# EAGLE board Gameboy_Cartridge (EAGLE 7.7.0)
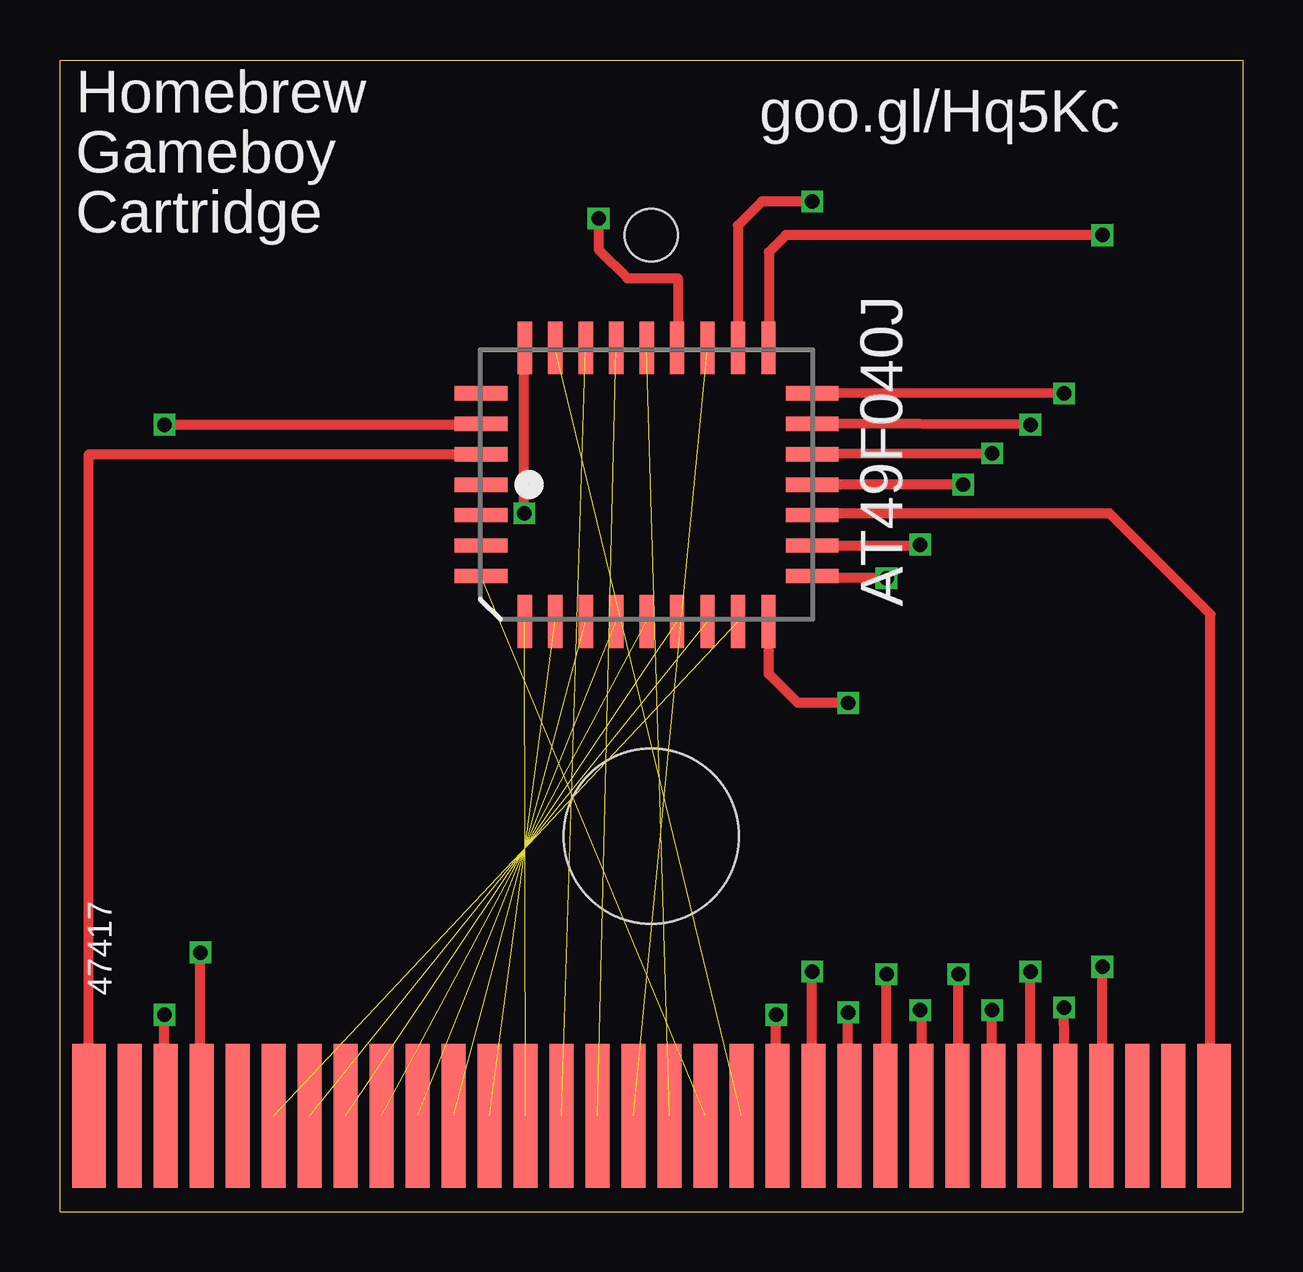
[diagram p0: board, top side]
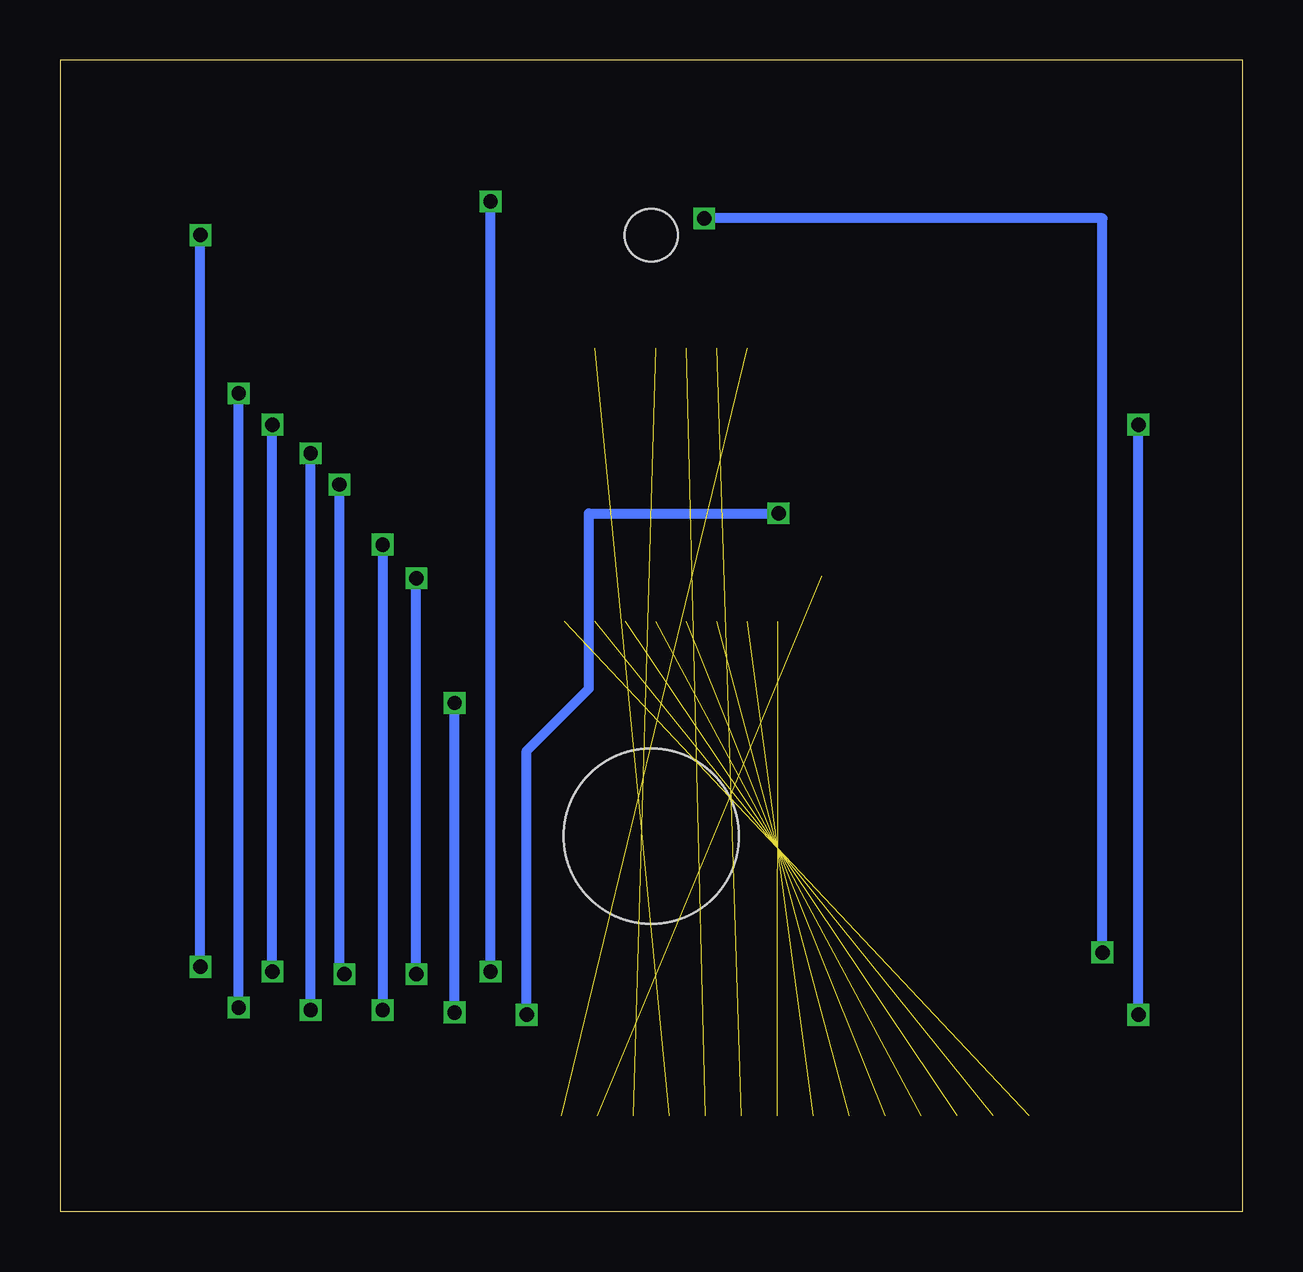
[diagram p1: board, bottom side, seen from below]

Size 49.3 x 48 mm. Coordinates in mm from the lower left corner, seen from the top.
Outline: 49.3,48 49.3,0 0,0 0,48 49.3,48
Copper layers (1*16): Top 0.035mm / dielectric 1.5mm / Bottom 0.035mm
Design rules "default": minimum track width 6mil, minimum drill 12mil, track to track 6mil, track to pad 6mil, pad to pad 6mil, via to via 6mil, smd to smd 0mil, copper to edge 10mil, drill to drill 10mil, minimum pad ring 10mil, minimum via ring 6mil, stop-mask expansion 2mil, vias tented up to drill 100mil, thermal gap 10mil
Holes 7.3 mm at 24.65,15.65
Holes 2.2 mm at 24.65,40.7

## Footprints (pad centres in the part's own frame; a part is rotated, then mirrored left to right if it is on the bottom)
PLCC32R = smd 0.6 x 2.2: 1 0,6.9; 2 -1.27,6.9; 3 -2.54,6.9; 4 -3.81,6.9; 14 -3.81,-6.9; 15 -2.54,-6.9; 16 -1.27,-6.9; 17 0,-6.9; 18 1.27,-6.9; 19 2.54,-6.9; 20 3.81,-6.9; 30 3.81,6.9; 31 2.54,6.9; 32 1.27,6.9 | smd 2.2 x 0.6: 5 -5.7,5.08; 6 -5.7,3.81; 7 -5.7,2.54; 8 -5.7,1.27; 9 -5.7,0; 10 -5.7,-1.27; 11 -5.7,-2.54; 12 -5.7,-3.81; 13 -5.7,-5.08; 21 5.7,-5.08; 22 5.7,-3.81; 23 5.7,-2.54; 24 5.7,-1.27; 25 5.7,0; 26 5.7,1.27; 27 5.7,2.54; 28 5.7,3.81; 29 5.7,5.08
CONNECTOR = smd 1.4 x 6: 1 0.7,-3; 32 47.6,-3 | smd 1 x 6: 2 2.4,-3; 3 3.9,-3; 4 5.4,-3; 5 6.9,-3; 6 8.4,-3; 7 9.9,-3; 8 11.4,-3; 9 12.9,-3; 10 14.4,-3; 11 15.9,-3; 12 17.4,-3; 13 18.9,-3; 14 20.4,-3; 15 21.9,-3; 16 23.4,-3; 17 24.9,-3; 18 26.4,-3; 19 27.9,-3; 20 29.4,-3; 21 30.9,-3; 22 32.4,-3; 23 33.9,-3; 24 35.4,-3; 25 36.9,-3; 26 38.4,-3; 27 39.9,-3; 28 41.4,-3; 29 42.9,-3; 30 44.4,-3; 31 45.9,-3

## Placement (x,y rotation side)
IC1  AT49F040J  [PLCC32R]  24.45,30.3 90 top
U$1  CONNECTOR  [CONNECTOR]  0.5,7 0 top

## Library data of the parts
IC1 U$1 = gameboy

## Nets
3: U$1.3
4: IC1.24 U$1.4
5: U$1.5
6: IC1.12 U$1.6
7: IC1.11 U$1.7
8: IC1.10 U$1.8
9: IC1.9 U$1.9
10: IC1.8 U$1.10
11: IC1.7 U$1.11
12: IC1.6 U$1.12
13: IC1.5 U$1.13
14: IC1.27 U$1.14
15: IC1.26 U$1.15
16: IC1.23 U$1.16
17: IC1.25 U$1.17
18: IC1.4 U$1.18
19: IC1.28 U$1.19
20: IC1.29 U$1.20
21: IC1.22 U$1.21
22: IC1.13 U$1.22
23: IC1.14 U$1.23
24: IC1.15 U$1.24
25: IC1.17 U$1.25
26: IC1.18 U$1.26
27: IC1.19 U$1.27
28: IC1.20 U$1.28
29: IC1.21 U$1.29
30: U$1.30
31: U$1.31
GND: IC1.16 U$1.32
S$1: IC1.31
VDD: IC1.32 U$1.1

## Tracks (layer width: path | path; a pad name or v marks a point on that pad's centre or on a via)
3  (via drill 0.6)
  Top 0.406: U$1.3 4.35,4 v4.35,8.2
  Bottom 0.406: v4.35,8.2 4.35,32.8
4  (via drill 0.6)
  Top 0.406: U$1.4 5.85,4 v5.85,10.8 | v22.45,41.4 22.45,40.1 23.65,38.9 25.75,38.9 25.75,36.03 IC1.24
  Bottom 0.406: v5.85,10.8 5.85,41.4 v22.45,41.4
6  (1 unrouted)
7  (1 unrouted)
8  (1 unrouted)
  Top 0.406: U$1.8 11.85,4
9  (1 unrouted)
10  (1 unrouted)
11  (1 unrouted)
12  (1 unrouted)
13  (1 unrouted)
14  (1 unrouted)
15  (1 unrouted)
16  (1 unrouted)
17  (1 unrouted)
18  (1 unrouted)
19  (1 unrouted)
20  (via drill 0.6)
  Top 0.406: U$1.20 29.85,4 v29.85,8.2 | v19.35,29.1 19.35,36 IC1.29
  Bottom 0.406: v29.85,8.2 29.85,19.2 27.25,21.8 27.25,29.1 v19.35,29.1
21  (via drill 0.6)
  Top 0.406: U$1.21 31.35,4 v31.35,10 | v31.35,42.1 29.25,42.1 28.25,41.1 IC1.22
  Bottom 0.406: v31.35,10 v31.35,42.1
22  (via drill 0.6)
  Top 0.406: U$1.22 32.85,4 v32.85,8.3 | v32.85,21.2 30.75,21.2 29.55,22.4 29.55,24.58 IC1.13
  Bottom 0.406: v32.85,8.3 v32.85,21.2
23  (via drill 0.6)
  Top 0.406: U$1.23 34.45,4 v34.45,9.9 | v34.45,26.4 31.35,26.4 IC1.14
  Bottom 0.406: v34.45,9.9 v34.45,26.4
24  (via drill 0.6)
  Top 0.406: IC1.15 35.85,27.76 v35.85,27.8 | v35.85,8.4 35.9,8.4 U$1.24
  Bottom 0.406: v35.85,27.8 v35.85,8.4
25  (via drill 0.6)
  Top 0.406: U$1.25 37.45,4 v37.45,9.9 | v37.65,30.3 IC1.17
  Bottom 0.406: v37.45,9.9 37.65,9.9 v37.65,30.3
26  (via drill 0.6)
  Top 0.406: U$1.26 38.85,4 v38.85,8.4 | v38.85,31.6 IC1.18
  Bottom 0.406: v38.85,8.4 v38.85,31.6
27  (via drill 0.6)
  Top 0.406: U$1.27 40.45,4 v40.45,10 | v40.45,32.8 IC1.19
  Bottom 0.406: v40.45,10 v40.45,32.8
28  (via drill 0.6)
  Top 0.406: U$1.28 v41.85,8.5 | v41.85,34.1 IC1.20
  Bottom 0.406: v41.85,8.5 v41.85,34.1
29  (via drill 0.6)
  Top 0.406: U$1.29 arc90 43.45,4.05 v43.45,10.2 | v43.45,40.7 30.25,40.7 29.55,40 29.55,36.02 IC1.21
  Bottom 0.406: v43.45,10.2 v43.45,40.7
GND
  Top 0.406: U$1.32 47.95,4 47.95,24.9 43.75,29.1 31.42,29.1 IC1.16
S$1  (via drill 0.6)
  Top 0.406: IC1.31 17.55,32.8 v4.35,32.8
VDD
  Top 0.406: U$1.1 1.2,31.57 IC1.32

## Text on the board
tPlace: Homebrew | goo.gl/Hq5Kc | Gameboy | Cartridge | 47417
